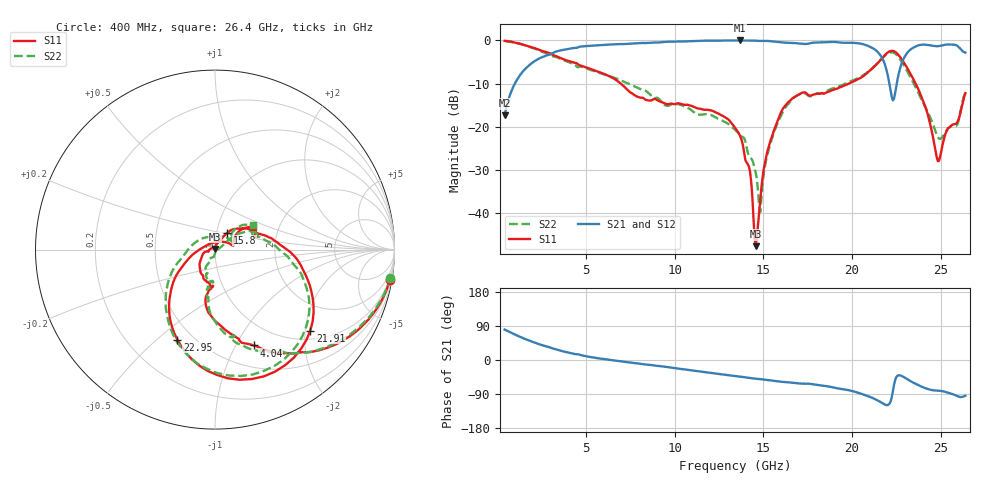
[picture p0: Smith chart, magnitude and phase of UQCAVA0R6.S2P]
!  Part Number  UQCAVA0R6
!  Description: RF capacitor  Mounting Orientation: Horizontal
!  Application:
# GHZ S DB R 50
! Freq  |S11|  S11 Ph  |S21|  S21 Ph  |S12|  S12 Ph  |S22|  S22 Ph
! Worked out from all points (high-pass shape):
!   401 points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, 400 MHz to 26.4 GHz, reference 50 ohm
!   highest |S21| = 0.00 dB at 13.66 GHz (marker M1); lowest = -17.3 dB at 400 MHz (marker M2)
!   |S21| within 3 dB of the highest: 3.07 GHz to 21.52 GHz (18.45 GHz wide, 150 % of centre); 23.09 GHz to end of sweep
!   lowest |S11| = -47.6 dB at 14.57 GHz (marker M3), VSWR 1.01, Z = 49.7 + j0.318 ohm
!   |S11| at or under -10 dB: 6.959 GHz to 19.82 GHz (12.86 GHz wide, 96 % of centre); 23.59 GHz to end of sweep
!   |S22| runs from -39.7 to -0.1 dB; largest |S21 - S12| = 0.0033
!   S11 on the Smith chart (normalised r, x): 400 MHz: 1, -12; 4.04 GHz: 0.74, -1.18; 15.8 GHz: 1.13, +0.22; 21.91 GHz: 1.22, -2.13; 22.95 GHz: 0.41, -0.58; 26.4 GHz: 1.47, +0.40
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0.4  -0.09 -9.8  -17.33 80.3  -17.34 80.3  -0.09 -9.1
1.635  -1.20 -35.8  -6.30 54.1  -6.31 54.1  -1.24 -35.3
4.04  -4.80 -68.1  -1.93 19.1  -1.93 19.2  -5.08 -73.7
4.755  -5.90 -75.9  -1.39 12.3  -1.40 12.4  -6.11 -79.9
9.11  -14.04 -98.4  -0.46 -15.8  -0.45 -15.7  -13.55 -100.8
13.4  -20.21 -144.4  -0.03 -42.2  -0.02 -42.2  -20.70 -116.9
13.66  -21.88 -153.5  0.00 -43.6  -0.01 -43.5  -21.75 -114.8
14.245  -30.33 179.2  -0.03 -47.4  -0.02 -47.4  -27.06 -104.2
14.57  -47.65 129.6  -0.08 -49.4  -0.07 -49.4  -30.63 -94.1
14.83  -36.44 83.7  -0.10 -50.4  -0.09 -50.4  -39.69 -20.5
15.155  -26.97 65.8  -0.10 -52.5  -0.09 -52.4  -27.75 25.1
15.805  -18.61 53.6  -0.34 -56.4  -0.33 -56.4  -19.13 35.8
17.755  -12.64 19.6  -0.55 -63.7  -0.54 -63.7  -12.80 25.8
20.55  -8.51 2.9  -0.79 -89.6  -0.78 -89.6  -8.28 -3.3
21.915  -3.14 -40.3  -6.33 -118.6  -6.32 -118.7  -3.29 -44.6
22.11  -2.55 -53.9  -9.97 -115.8  -9.95 -115.8  -2.82 -58.1
22.37  -2.50 -74.1  -13.54 -66.3  -13.53 -66.5  -2.87 -78.5
22.955  -5.30 -112.7  -3.92 -45.9  -3.90 -46.0  -5.98 -119.8
23.865  -12.49 -148.8  -1.02 -69.0  -1.00 -69.0  -13.21 -160.9
24.84  -27.93 115.5  -1.33 -80.8  -1.31 -81.0  -22.38 113.9
25.88  -19.29 18.7  -1.09 -94.0  -1.08 -94.1  -19.79 31.1
26.4  -12.20 31.0  -2.81 -94.2  -2.80 -94.3  -11.96 32.6
